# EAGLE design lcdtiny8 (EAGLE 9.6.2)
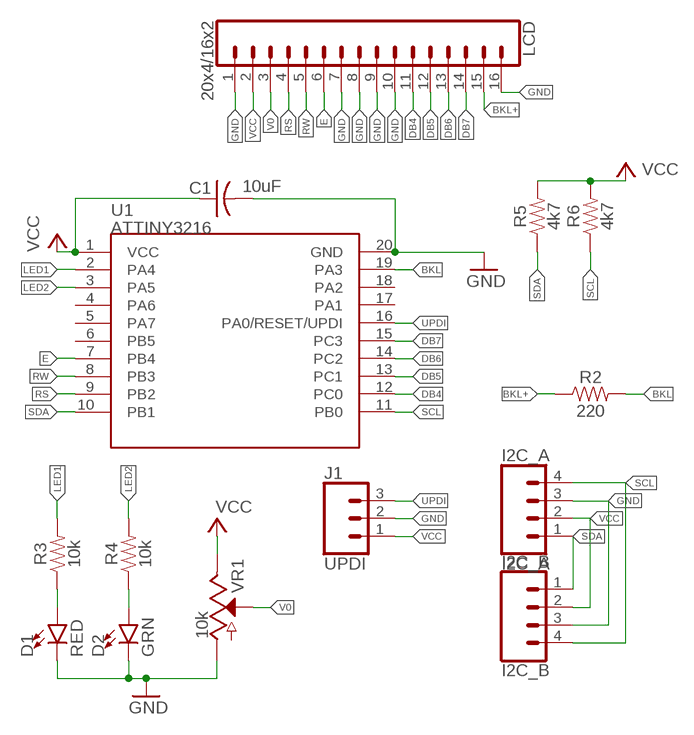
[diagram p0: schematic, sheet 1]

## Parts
C1  10uF  C-US050-025X075  [C050-025X075]
D1  RED  LED3MM  [LED_3MM]
D2  GRN  LED3MM  [LED_3MM]
I2C_A  I2C_A  CONN_04JST-PTH-VERT  [JST-4-PTH-VERT]
I2C_B  I2C_B  CONN_04JST-PTH-VERT  [JST-4-PTH-VERT]
J1  UPDI  CONN_03JST-PTH-VERT  [JST-3-PTH-VERT]
LCD  20x4/16x2  CONN_16  [1X16]
R2  220  330OHM-HORIZ-1/10W-5%  [AXIAL-0.3]
R3  10k  10KOHM-HORIZ-1/6W-5%  [AXIAL-0.3]
R4  10k  10KOHM-HORIZ-1/6W-5%  [AXIAL-0.3]
R5  4k7  330OHM-HORIZ-1/10W-5%  [AXIAL-0.3]
R6  4k7  330OHM-HORIZ-1/10W-5%  [AXIAL-0.3]
U1  ATTINY3216  [SOP20W]
VR1  10k  POTENTIOMETER-PTH-9MM-1/20W-20%  [POT-PTH-ALPS]

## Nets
BKL: R2.P$2 U1.19(PA3)
BKL+: LCD.15 R2.P$1
DB4: LCD.11 U1.12(PC0)
DB5: LCD.12 U1.13(PC1)
DB6: LCD.13 U1.14(PC2)
DB7: LCD.14 U1.15(PC3)
E: LCD.6 U1.7(PB4)
GND: C1.2 D1.K(C) D2.K(C) I2C_A.3 I2C_B.3 J1.2 LCD.1 LCD.7 LCD.8 LCD.9 LCD.10 LCD.16 U1.20(GND) VR1.P$3(A)
LED1: R3.P$2 U1.2(PA4)
LED2: R4.P$2 U1.3(PA5)
N$1: D1.A R3.P$1
N$2: D2.A R4.P$1
RS: LCD.4 U1.9(PB2)
RW: LCD.5 U1.8(PB3)
SCL: I2C_A.4 I2C_B.4 R6.P$1 U1.11(PB0)
SDA: I2C_A.1 I2C_B.1 R5.P$1 U1.10(PB1)
UPDI: J1.3 U1.16(PA0/RESET/UPDI)
V0: LCD.3 VR1.P$2(S)
VCC: C1.1 I2C_A.2 I2C_B.2 J1.1 LCD.2 R5.P$2 R6.P$2 U1.1(VCC) VR1.P$1(E)
Unconnected: U1.4(PA6) U1.5(PA7) U1.6(PB5) U1.17(PA1) U1.18(PA2)

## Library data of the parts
C1 = adafruit:C-US: CAPACITOR, American symbol
D1 D2 = SparkFun-LED:LED: LED (Generic); PROD_ID: DIO-08794
I2C_A I2C_B = SparkFun-Connectors:CONN_04: Multi connection point. Often used as Generic Header-pin footprint for 0.1 inch spaced/style header connections On any of the 0.1 inch spaced packages, you can populate with these: Break Away Headers - Straight (PRT-00116) Break Away Male Headers - Right Angle (PRT-00553) Female Headers (PRT-00115)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; PROD_ID: CONN-13251
J1 = SparkFun-Connectors:CONN_03: Multi connection point. Often used as Generic Header-pin footprint for 0.1 inch spaced/style header connections On any of the 0.1 inch spaced packages, you can populate with these: Break Away Headers - Straight (PRT-00116) Break Away Male Headers - Right Angle (PRT-00553) Female Headers (PRT-00115)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; PROD_ID: CONN-13230
LCD = SparkFun-Connectors:CONN_16: Multi connection point. Often used as Generic Header-pin footprint for 0.1 inch spaced/style header connections On any of the 0.1 inch spaced packages, you can populate with these: Break Away Headers - Straight (PRT-00116) Break Away Male Headers - Right Angle (PRT-00553) Female Headers (PRT-00115)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
R2 R5 R6 = SparkFun-Resistors:330OHM: 330Ω resistor; PROD_ID: RES-8371; VALUE: 330
R3 R4 = SparkFun-Resistors:10KOHM: 10kΩ resistor; PROD_ID: RES-08375
U1 = seebs-bits:ATTINY3216: ATTINY3216 32kB 20MHz I2C/SPI/UART
VR1 = SparkFun-Resistors:POTENTIOMETER: Potentiometer (Pot) Three-terminal potentiometers, with an adjustable wiper and two adjustable resistors. A pot can be used to create a configurable voltage divider, or as a variable resistor. Variants ALPS_POT and ALPS_POT_KIT - PTH, breadboard compatible, 9mm square pots Rotary Potentiometer -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; PROD_ID: RES-09177; SF_SKU: COM-09288

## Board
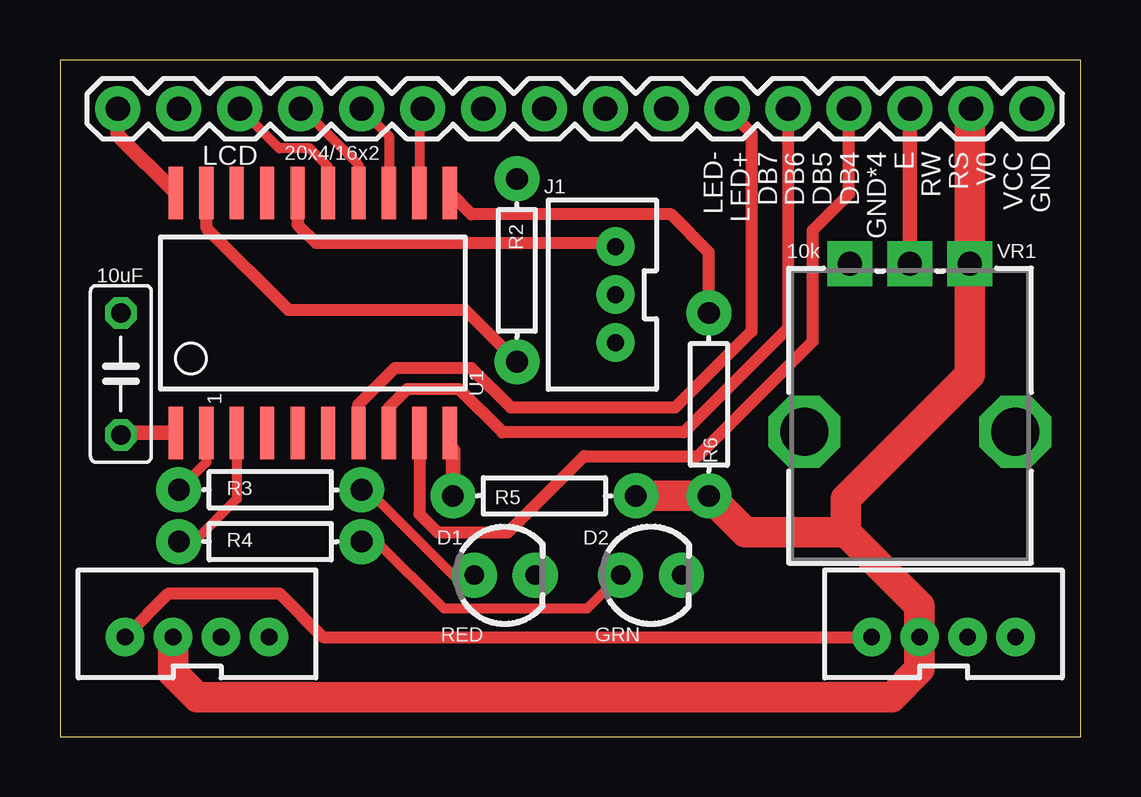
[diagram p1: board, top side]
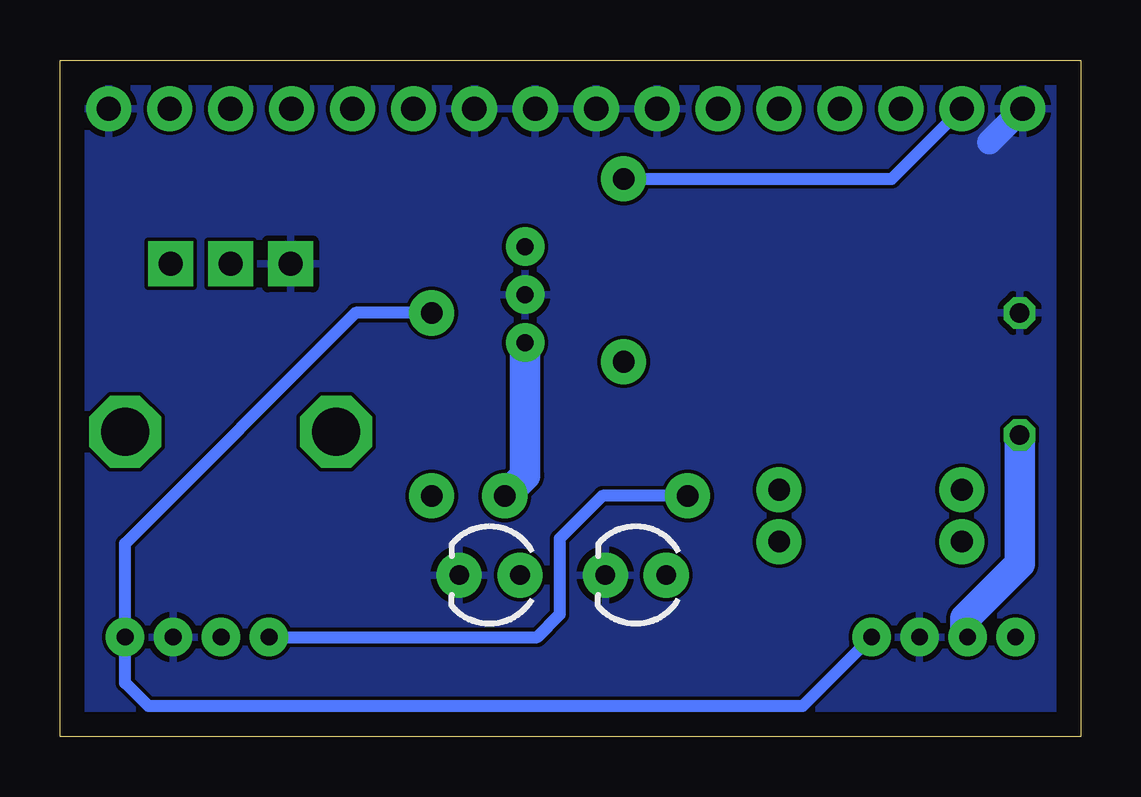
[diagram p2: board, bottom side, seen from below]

Size 42.55 x 28.19 mm. Coordinates in mm from the lower left corner, seen from the top.
Outline: 0,0 42.55,0 42.55,28.19 0,28.19 0,0
Copper layers (1*16): Top 0.035mm / dielectric 1.5mm / Bottom 0.035mm
Design rules "conservative": minimum track width 8mil, minimum drill 0.35mm, track to track 6mil, track to pad 6mil, pad to pad 6mil, via to via 6mil, smd to smd 6mil, copper to edge 40mil, drill to drill 6mil, minimum pad ring 10mil, minimum via ring 8mil, stop-mask expansion 4mil, vias tented up to drill 0mil, thermal gap 10mil

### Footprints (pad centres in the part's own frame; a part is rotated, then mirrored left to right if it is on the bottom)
C050-025X075 = drill 0.813 octagon: 1 -2.54,0; 2 2.54,0
LED_3MM = drill 0.813 pad 1.88: A -1.27,0; K 1.27,0
JST-4-PTH-VERT = drill 0.7 pad 1.6: 1 -3,-0.55; 2 -1,-0.55; 3 1,-0.55; 4 3,-0.55
JST-3-PTH-VERT = drill 0.7 pad 1.6: 1 -2,-0.55; 2 0,-0.55; 3 2,-0.55
1X16 = drill 1.016 pad 1.88: 1 0,0; 2 2.54,0; 3 5.08,0; 4 7.62,0; 5 10.16,0; 6 12.7,0; 7 15.24,0; 8 17.78,0; 9 20.32,0; 10 22.86,0; 11 25.4,0; 12 27.94,0; 13 30.48,0; 14 33.02,0; 15 35.56,0; 16 38.1,0
AXIAL-0.3 = drill 0.9 pad 1.88: P$1 -3.81,0; P$2 3.81,0
SOP20W = smd 0.6 x 2.2: 1 -5.715,-5; 2 -4.445,-5; 3 -3.175,-5; 4 -1.905,-5; 5 -0.635,-5; 6 0.635,-5; 7 1.905,-5; 8 3.175,-5; 9 4.445,-5; 10 5.715,-5; 11 5.715,5; 12 4.445,5; 13 3.175,5; 14 1.905,5; 15 0.635,5; 16 -0.635,5; 17 -1.905,5; 18 -3.175,5; 19 -4.445,5; 20 -5.715,5
POT-PTH-ALPS = drill 1 pad 1.88 square: P$1 7,-2.5; P$2 7,0; P$3 7,2.5 | drill 2 octagon: P$4 0,-4.4; P$5 0,4.4

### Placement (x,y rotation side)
C1  2.54,15.11 90 top
D1  18.54,6.73 0 top
D2  24.64,6.73 0 top
I2C_A  5.71,4.7 0 top
I2C_B  36.83,4.7 0 top
J1  22.61,18.41 90 top
LCD  40.51,26.16 180 top
R2  19.05,19.43 270 top
R3  8.76,10.29 180 top
R4  8.76,8.13 180 top
R5  20.19,10.03 0 top
R6  27.05,13.84 270 top
U1  10.54,17.65 0 top
VR1  35.43,12.7 90 top

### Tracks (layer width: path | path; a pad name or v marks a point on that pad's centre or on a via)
BKL
  Top 0.508: U1.19 6.1,21.21 9.53,17.78 16.89,17.78 R2.P$2
BKL+
  Bottom 0.508: R2.P$1 7.87,23.24 LCD.15
DB4
  Top 0.406: LCD.11 14.99,26.04 U1.12
DB5
  Top 0.406: LCD.12 13.72,25.02 U1.13
DB6
  Top 0.406: LCD.13 10.11,26.16 12.45,23.82 U1.14
DB7
  Top 0.406: LCD.14 9.14,24.51 10.41,24.51 11.18,23.75 U1.15
E
  Top 0.508: U1.7 12.45,13.84 13.97,15.37 17.14,15.37 18.8,13.72 25.65,13.72 28.83,16.89 28.83,25.15 LCD.6
GND
  Top 0.61: U1.20 2.41,25.07 LCD.16
  Bottom 1.016: 3.81,24.77 LCD.16
  pour Bottom: 0,28.19 42.55,28.19 42.55,0 0,0
LED1
  Top 0.406: R3.P$2 6.1,11.43 U1.2
LED2
  Top 0.406: U1.3 7.37,9.91 5.59,8.13 R4.P$2
N$1
  Top 0.406: D1.A 16.38,6.73 12.83,10.29 R3.P$1
N$2
  Top 0.406: D2.A 21.97,5.33 16,5.33 13.21,8.13 R4.P$1
RS
  Top 0.508: LCD.4 32.89,22.61 31.37,21.08 31.37,16.45 26.6,11.68 21.84,11.68 18.67,8.51 15.75,8.51 14.99,9.27 U1.9
RW
  Top 0.508: U1.8 13.72,13.72 14.48,14.48 16.64,14.48 18.44,12.68 26.01,12.68 30.35,17.02 LCD.5
SCL
  Top 0.508: R6.P$1 27.05,20.19 25.48,21.76 17.14,21.76 U1.11
  Bottom 0.508: R6.P$1 30.22,17.65 39.83,8.05 I2C_B.4 39.83,2.24 38.86,1.27 11.59,1.27 I2C_A.4
SDA
  Top 0.508: I2C_A.1 4.54,5.97 9.15,5.97 10.97,4.15 I2C_B.1
  Top 0.61: R5.P$1 16.38,11.94 16.26,12.06 U1.10
  Bottom 0.508: R5.P$1 19.94,10.03 21.72,8.26 21.72,5.08 22.65,4.15 I2C_B.1
UPDI
  Top 0.508: U1.16 9.91,21.34 10.67,20.57 23,20.57 J1.3
V0
  Top 0.61: LCD.3 VR1.P$2
VCC
  Top 0.61: U1.1 2.62,12.65 C1.1
  Top 1.27: LCD.2 37.93,26.12 VR1.P$1 37.93,15.07 32.77,9.91 32.77,8.51 | I2C_A.2 4.71,2.65 5.71,1.65 34.67,1.65 35.83,2.81 I2C_B.2 35.83,5.45 32.77,8.51 | 32.77,8.51 28.58,8.51 R6.P$2 R5.P$2
  Bottom 1.27: I2C_A.2 4.81,4.24 4.81,4.93 2.54,7.2 C1.1 | R5.P$2 23.16,10.88 J1.1

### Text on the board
tSilk: 1
_tsilk: LED- / LED+ / DB7 / DB6 / DB5 / DB4 / GND*4 / E / RW / RS / V0 / VCC / GND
